(* Logix 5000 AddOnInstructionDefinition export LogixAI_AutoTrainCal_AOI; software revision 32.00 *)

TYPE LogixAI_Calculations :
STRUCT
   Success : DINT;
   ActualValue : REAL;
   PredictedValue : REAL;
   RelativeError : REAL;
   AnomalyDetected : DINT;
END_STRUCT
END_TYPE

TYPE LogixAI_Training :
STRUCT
   AbsoluteError : REAL;
   RelativeError : REAL;
   Confidence : REAL;
END_STRUCT
END_TYPE

TYPE TrainPredictDummytDataType :
STRUCT
   State : DINT;
   Calculate : DINT;
   SmartTrain : DINT;
   Train : DINT;
   ForceTraining : DINT;
   FaultCode : DINT;
   Calculations : LogixAI_Calculations;
   Training : LogixAI_Training;
END_STRUCT
END_TYPE

ADD_ON_INSTRUCTION LogixAI_AutoTrainCal_AOI   (* revision 1.0, ExecutePrescan *)
VAR_IN_OUT
   Model_Tags : TrainPredictDummytDataType; {required}
END_VAR
VAR_INPUT
   Set_AutoTrainCycles : DINT; {visible}
   Cmd_AutoTrain : BOOL; {visible}
   Cmd_SingleTrain : BOOL;
   Cmd_AutoCalculate : BOOL; {visible}
   Cmd_SingleCalculate : BOOL;
   Cmd_Stop : BOOL; {visible}
END_VAR
VAR_OUTPUT
   Sts_Training : BOOL; {access Read Only}
   Sts_AutoCalculate : BOOL; {access Read Only, visible}
   Sts_AutoTraining : BOOL; {access Read Only, visible}
   Sts_AutoTrainDone : BOOL; {access Read Only, visible}
   Val_AutoTrainCycles : DINT; {access Read Only, visible}
   Val_AutoTrainCount : DINT; {access Read Only, visible}
   Val_Confidence : REAL; {access Read Only, visible}
   Val_PredictedValue : REAL; {access Read Only, visible}
   Val_ActualValue : REAL; {access Read Only, visible}
   Val_TrainCount : DINT; {access Read Only}
   Val_Error : REAL; {access Read Only}
END_VAR
VAR
   pCmd_SingleTrain : BOOL; {access None}
   pCmd_AutoTrain : BOOL; {access None}
   pCmd_SingleCalculate : BOOL; {access None}
   pCmd_AutoCalculate : BOOL; {access None}
   pAutoTrain_Index : DINT; {access None}
   ONS : DINT; {access None}
END_VAR

ROUTINE Logic   (* ladder *)
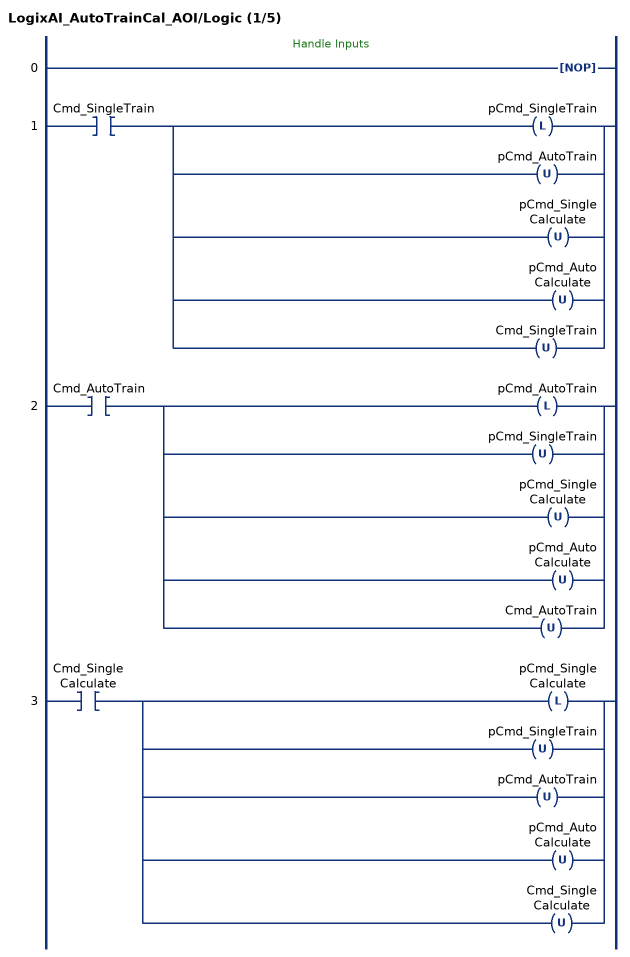
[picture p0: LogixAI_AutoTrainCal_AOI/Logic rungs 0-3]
   // Handle Inputs
   0: NOP();
   1: XIC(Cmd_SingleTrain)[OTL(pCmd_SingleTrain) ,OTU(pCmd_AutoTrain) ,OTU(pCmd_SingleCalculate) ,OTU(pCmd_AutoCalculate) ,OTU(Cmd_SingleTrain) ];
   2: XIC(Cmd_AutoTrain)[OTL(pCmd_AutoTrain) ,OTU(pCmd_SingleTrain) ,OTU(pCmd_SingleCalculate) ,OTU(pCmd_AutoCalculate) ,OTU(Cmd_AutoTrain) ];
   3: XIC(Cmd_SingleCalculate)[OTL(pCmd_SingleCalculate) ,OTU(pCmd_SingleTrain) ,OTU(pCmd_AutoTrain) ,OTU(pCmd_AutoCalculate) ,OTU(Cmd_SingleCalculate) ];
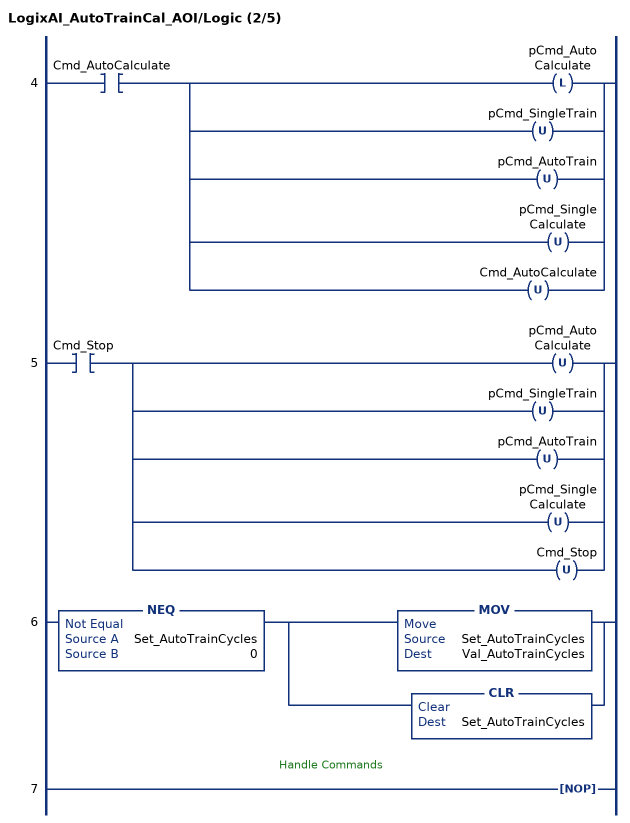
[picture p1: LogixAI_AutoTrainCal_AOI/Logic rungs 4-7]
   4: XIC(Cmd_AutoCalculate)[OTL(pCmd_AutoCalculate) ,OTU(pCmd_SingleTrain) ,OTU(pCmd_AutoTrain) ,OTU(pCmd_SingleCalculate) ,OTU(Cmd_AutoCalculate) ];
   5: XIC(Cmd_Stop)[OTU(pCmd_AutoCalculate) ,OTU(pCmd_SingleTrain) ,OTU(pCmd_AutoTrain) ,OTU(pCmd_SingleCalculate) ,OTU(Cmd_Stop) ];
   6: NEQ(Set_AutoTrainCycles,0)[MOV(Set_AutoTrainCycles,Val_AutoTrainCycles) ,CLR(Set_AutoTrainCycles) ];
   // Handle Commands
   7: NOP();
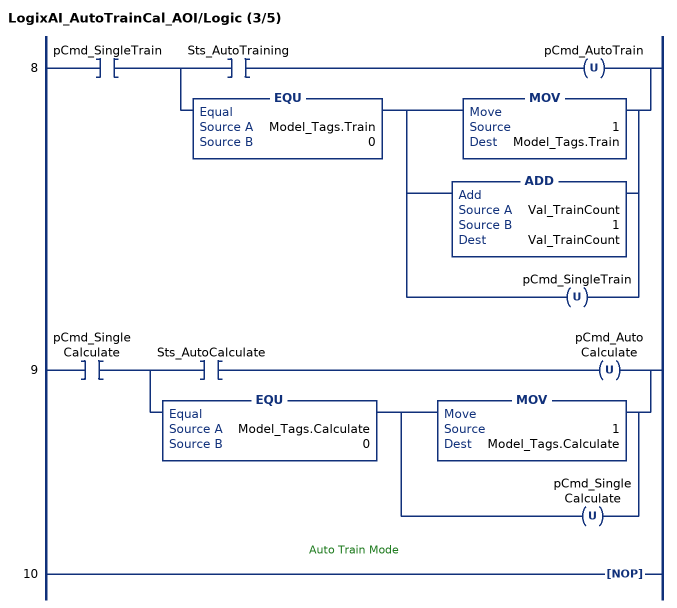
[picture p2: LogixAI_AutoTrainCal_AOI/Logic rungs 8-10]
   8: XIC(pCmd_SingleTrain)[XIC(Sts_AutoTraining) OTU(pCmd_AutoTrain) ,EQU(Model_Tags.Train,0) [MOV(1,Model_Tags.Train) ,ADD(Val_TrainCount,1,Val_TrainCount) ,OTU(pCmd_SingleTrain) ] ];
   9: XIC(pCmd_SingleCalculate)[XIC(Sts_AutoCalculate) OTU(pCmd_AutoCalculate) ,EQU(Model_Tags.Calculate,0) [MOV(1,Model_Tags.Calculate) ,OTU(pCmd_SingleCalculate) ] ];
   // Auto Train Mode
   10: NOP();
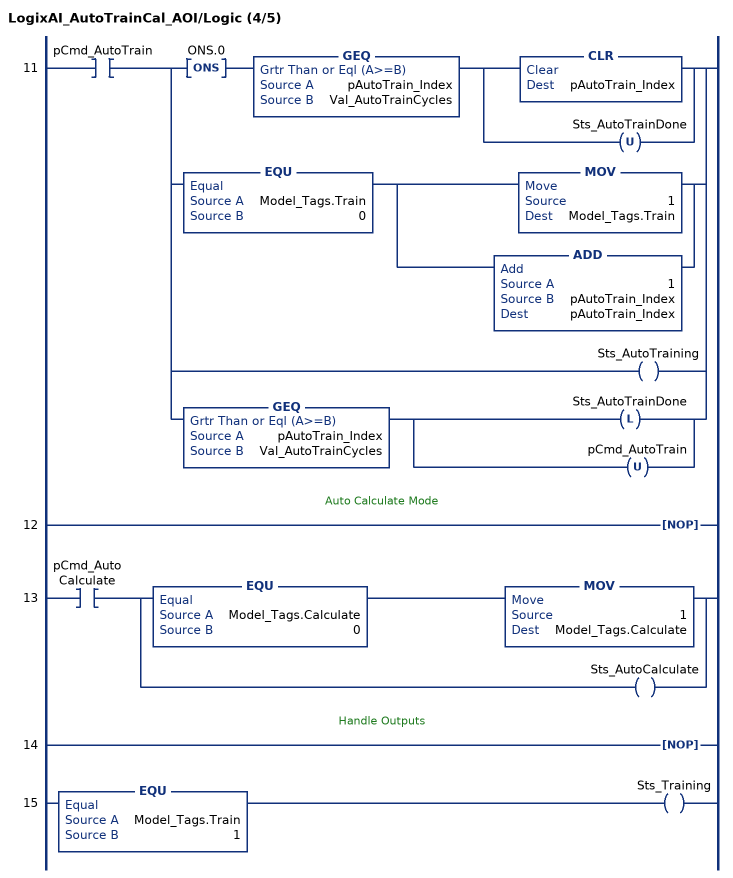
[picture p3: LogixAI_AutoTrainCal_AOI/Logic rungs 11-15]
   11: XIC(pCmd_AutoTrain)[ONS(ONS.0) GEQ(pAutoTrain_Index,Val_AutoTrainCycles) [CLR(pAutoTrain_Index) ,OTU(Sts_AutoTrainDone) ] ,EQU(Model_Tags.Train,0) [MOV(1,Model_Tags.Train) ,ADD(1,pAutoTrain_Index,pAutoTrain_Index) ] ,OTE(Sts_AutoTraining) ,GEQ(pAutoTrain_Index,Val_AutoTrainCycles) [OTL(Sts_AutoTrainDone) ,OTU(pCmd_AutoTrain) ] ];
   // Auto Calculate Mode
   12: NOP();
   13: XIC(pCmd_AutoCalculate)[EQU(Model_Tags.Calculate,0) MOV(1,Model_Tags.Calculate) ,OTE(Sts_AutoCalculate) ];
   // Handle Outputs
   14: NOP();
   15: EQU(Model_Tags.Train,1)OTE(Sts_Training);
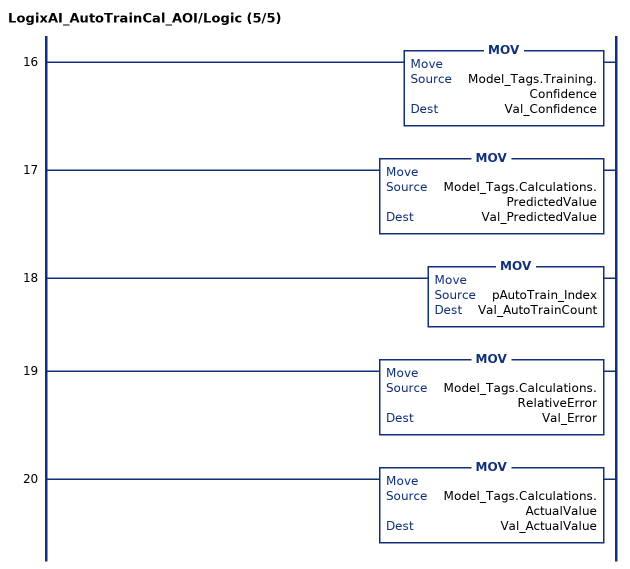
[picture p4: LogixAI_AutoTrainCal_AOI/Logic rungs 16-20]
   16: MOV(Model_Tags.Training.Confidence,Val_Confidence);
   17: MOV(Model_Tags.Calculations.PredictedValue,Val_PredictedValue);
   18: MOV(pAutoTrain_Index,Val_AutoTrainCount);
   19: MOV(Model_Tags.Calculations.RelativeError,Val_Error);
   20: MOV(Model_Tags.Calculations.ActualValue,Val_ActualValue);
END_ROUTINE

ROUTINE Prescan   (* ladder *)
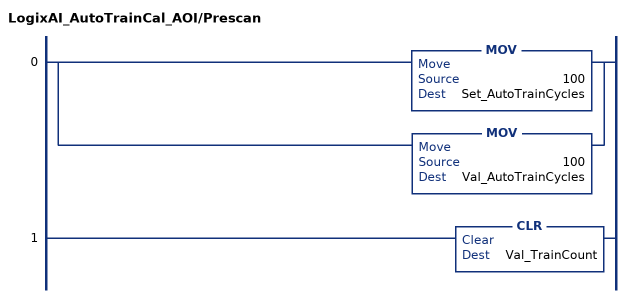
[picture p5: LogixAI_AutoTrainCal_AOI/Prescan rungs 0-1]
   0: [MOV(100,Set_AutoTrainCycles) ,MOV(100,Val_AutoTrainCycles) ];
   1: CLR(Val_TrainCount);
END_ROUTINE
END_ADD_ON_INSTRUCTION
